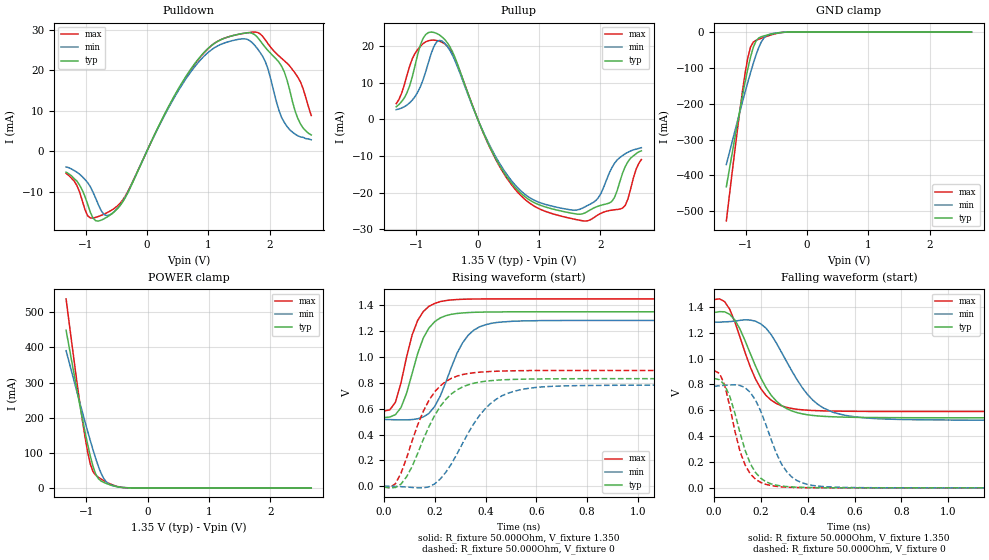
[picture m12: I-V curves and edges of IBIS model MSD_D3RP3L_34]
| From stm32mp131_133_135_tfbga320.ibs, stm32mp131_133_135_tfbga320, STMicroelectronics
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[Model] MSD_D3RP3L_34
Model_type   I/O
C_comp 2.240pF   2.158pF   2.357pF
Vinh = 810.000mV
Vinl = 540.000mV
Vmeas = 675.000mV
Vref = 675.000mV
[Model Spec]
Vinh   810.000mV   777.000mV   860.000mV
Vinl   540.000mV   507.000mV   590.000mV
Vmeas   675.000mV   642.000mV   725.000mV
Vref   675.000mV   642.000mV   725.000mV
[Receiver Thresholds]
Vth   =  0.675V
Vth_min  =  0.6615V
Vth_max  =  0.6885V
Vinh_ac  =  0.160V
Vinh_dc  =  0.090V
Vinl_ac  = -0.160V
Vinl_dc  = -0.090V
Tslew_ac =  5.000ns |Not specified, so set to high value
Threshold_sensitivity = 0.50
Reference_supply Pullup_ref
[Temperature Range]   25.000   125.000   -40.000
[Voltage Range]   1.350V   1.283V   1.450V
[GND Clamp Reference]   0.00V   0.00V   0.00V
[Pulldown Reference]   0.00V   0.00V   0.00V
[POWER Clamp Reference]   1.350V   1.283V   1.450V
[Pullup Reference]   1.350V   1.283V   1.450V
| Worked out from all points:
|   slope of the pulldown table from 0 to 0.203 V, typ, clamps not added: 31 ohm
|   slope of the pullup table from 0 to 0.203 V, typ, clamps not added: 26.2 ohm
|   GND clamp passes 1 mA (typ) near -0.41 V on its own axis
|   POWER clamp passes 1 mA (typ) near -0.41 V on its own axis
|   rising waveform, R_fixture 50.000Ohm, V_fixture 1.350: 20-80 % time 81.9ps typ, 103ps min, 70.8ps max; typ from 0.532 V to 1.35 V
|   rising waveform, R_fixture 50.000Ohm, V_fixture 0: 20-80 % time 128ps typ, 152ps min, 114ps max; typ from -0.007 V to 0.832 V
|   falling waveform, R_fixture 50.000Ohm, V_fixture 1.350: 20-80 % time 130ps typ, 161ps min, 112ps max; typ from 1.36 V to 0.542 V
|   falling waveform, R_fixture 50.000Ohm, V_fixture 0: 20-80 % time 88.3ps typ, 108ps min, 77ps max; typ from 0.846 V to 0 V
[GND Clamp]
-1.318V   -432mA     -369.8mA   -527.4mA
-1.142V   -260.2mA   -252.4mA   -279.5mA
-1.055V   -177.9mA   -195mA     -164.8mA
-1.011V   -138.8mA   -167mA     -113.9mA
-966.7mV  -102.2mA   -139.6mA   -71.13mA
-922.7mV  -69.41mA   -113.1mA   -41.59mA
-878.8mV  -42.86mA   -87.83mA   -28.26mA
-790.9mV  -16.84mA   -43.84mA   -20.19mA
-703mV    -10.77mA   -15.97mA   -14.59mA
-527.3mV  -3.881mA   -3.286mA   -5.179mA
-263.6mV  -34.33uA   -68.91uA   -22.73uA
2.68V     23.23nA    650.7nA    2.895nA
[Power Clamp]
-1.33V    448.9mA    390.9mA    538.4mA
-1.111V   240.1mA    246mA      248.4mA
-1.023V   161.2mA    189.4mA    146.7mA
-978.8mV  124.3mA    161.6mA    102.6mA
-934.9mV  90.54mA    134.5mA    67.58mA
-890.9mV  61.4mA     108.3mA    46.23mA
-847mV    39.26mA    83.52mA    35.86mA
-803mV    26.02mA    60.85mA    29.84mA
-715.1mV  15.45mA    26.31mA    20.45mA
-671.2mV  12.26mA    16.27mA    16.34mA
-407.6mV  879.8uA    1.157mA    1.067mA
2.668V    -39.9nA    -766.6nA   -3.595nA
[Pulldown]
-1.318V   -5.2mA     -3.9mA     -5.5mA
-922.7mV  -15.09mA   -8.8mA     -16.52mA
-703mV    -16.76mA   -15.61mA   -15.61mA
-571.2mV  -15.49mA   -15.45mA   -14.56mA
-351.5mV  -11.47mA   -11.32mA   -11.1mA
747mV     20.94mA    20.22mA    20.78mA
1.142V    27.04mA    25.92mA    27.06mA
1.626V    29.25mA    27.69mA    29.23mA
1.933V    25.6mA     22.07mA    27.47mA
2.241V    19.58mA    7.1mA      22.34mA
2.461V    8.1mA      3.8mA      18.3mA
2.68V     4mA        2.8mA      8.8mA
[Pullup]
-1.33V    3.4mA      2.605mA    4.252mA
-1.155V   7.2mA      3.862mA    11.96mA
-978.8mV  17.7mA     7.382mA    19.01mA
-715.1mV  23.64mA    19.82mA    21.55mA
-451.5mV  19.66mA    18.67mA    18.98mA
251.5mV   -9.371mA   -8.922mA   -9.594mA
866.7mV   -22.21mA   -21.56mA   -23.09mA
1.702V    -25.79mA   -24.26mA   -27.63mA
1.965V    -23.66mA   -21.42mA   -26mA
2.185V    -22.39mA   -13.25mA   -24.76mA
2.361V    -14.7mA    -9.885mA   -24.21mA
2.668V    -8.6mA     -7.748mA   -10.98mA
[Ramp]
R_load=50.000Ohm
dV/dt_r   492.090mV/103.500ps  462.629mV/126.500ps  526.560mV/91.500ps
dV/dt_f   492.090mV/108.500ps  462.629mV/134.500ps  526.560mV/94.500ps
[Rising waveform]
R_fixture=50.000Ohm
V_fixture=1.350
V_fixture_min=1.283
V_fixture_max=1.450
0s        531.8mV    517.2mV    582.6mV
45ps      553.6mV    514.3mV    648.9mV
67ps      608mV      513.4mV    799mV
133ps     1.028V     522.1mV    1.284V
177ps     1.224V     563.7mV    1.392V
222ps     1.303V     699.4mV    1.429V
288ps     1.337V     1.03V      1.445V
332ps     1.344V     1.169V     1.448V
443ps     1.349V     1.267V     1.45V
2.167ns   1.35V      1.283V     1.45V
[Rising waveform]
R_fixture=50.000Ohm
V_fixture=0
0s        -6.851mV   775.2uV    -6.466mV
45ps      -9.722mV   -1.181mV   19.08mV
89ps      72.69mV    -6.064mV   217.9mV
155ps     362.2mV    -12.39mV   580.1mV
200ps     549.6mV    18.55mV    731mV
244ps     673.5mV    109.2mV    810.9mV
310ps     768.7mV    333mV      864.3mV
421ps     817.2mV    642.1mV    888.1mV
576ps     829.4mV    759.3mV    895mV
2.167ns   832.4mV    782.4mV    896mV
[Falling waveform]
R_fixture=50.000Ohm
V_fixture=1.350
V_fixture_min=1.283
V_fixture_max=1.450
0s        1.357V     1.282V     1.456V
45ps      1.362V     1.284V     1.441V
89ps      1.298V     1.29V      1.282V
155ps     1.038V     1.298V     933.9mV
200ps     850.3mV    1.268V     766.8mV
244ps     715.7mV    1.185V     678mV
310ps     613mV      976.6mV    622.5mV
443ps     556.3mV    646.1mV    597mV
598ps     545.7mV    550.3mV    592mV
2.167ns   542.1mV    523.3mV    590.8mV
[Falling waveform]
R_fixture=50.000Ohm
V_fixture=0
0s        845.7mV    786.1mV    905.7mV
45ps      796.4mV    793.2mV    797.1mV
67ps      708.9mV    796.4mV    631.2mV
111ps     424.9mV    792mV      280.5mV
133ps     288.2mV    774.4mV    174.7mV
177ps     118.6mV    679.1mV    66.44mV
244ps     30.47mV    373mV      17.43mV
332ps     7.048mV    83.94mV    3.414mV
443ps     1.423mV    13.74mV    424.6uV
2.167ns   0V         2.128uV    0V
